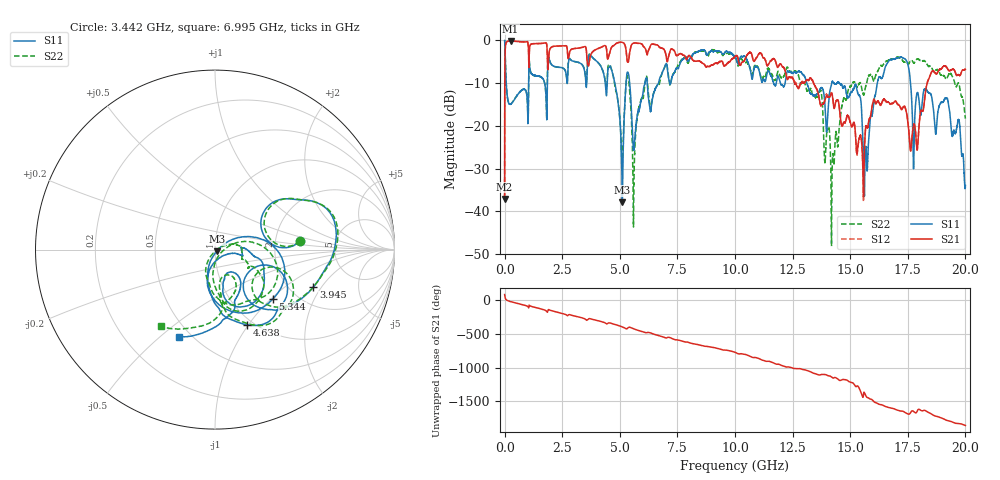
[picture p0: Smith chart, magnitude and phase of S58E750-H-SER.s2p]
!{S58E750}
!Johanson Technology Inc.
!www.johansontechnology.com
!Test Board Conditions:
!Substrate Type  RO4350B
!Substrate Thickness  60 mil
!Substrate Dk  3.66
!TL Type: GCPW
!TL Trace Width  115 mil
!TL Gap  52 mil
!Electrode orientation  Horizontal
!DUT TOPOLOGY	SERIES
!Mounting Pad LxW  55x428 mil
! Created Wed Apr 14 12:01:42 2021
# mhz S ma R 50
! 2 Port Network Data from SP1.SP block
! freq  magS11  angS11  magS21  angS21  magS12  angS12  magS22  angS22
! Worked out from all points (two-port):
!   20001 points, 300 kHz to 20 GHz, reference 50 ohm
!   highest |S21| = -0.15 dB at 256.3 MHz (marker M1); lowest = -37.2 dB at 300 kHz (marker M2)
!   |S21| within 3 dB of the highest: 21.1 MHz to 1.042 GHz (1.021 GHz wide, 192 % of centre); 1.925 GHz to 2.731 GHz (805.9 MHz wide, 34.6 % of centre)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
!   lowest |S11| = -37.9 dB at 5.11 GHz (marker M3), VSWR 1.03, Z = 51 - j0.854 ohm
!   |S11| at or under -10 dB: 13.12 GHz to 14.2 GHz (1.082 GHz wide, 7.92 % of centre); 14.54 GHz to 16.18 GHz (1.641 GHz wide, 10.7 % of centre); 17.62 GHz to end of sweep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
!   |S22| runs from -48.2 to 0.0 dB; largest |S21 - S12| = 0.016
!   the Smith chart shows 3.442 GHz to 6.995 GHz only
!   S11 on the Smith chart (normalised r, x): 3.442 GHz: 2.75, +0.35; 3.945 GHz: 2.64, -1.69; 4.638 GHz: 0.93, -0.99; 5.344 GHz: 1.54, -1.03; 6.995 GHz: 0.43, -0.58
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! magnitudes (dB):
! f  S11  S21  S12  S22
! 300 kHz  0.0  -37.2  -37.1  -0.1
! 104.3 MHz  -12.5  -0.3  -0.3  -12.5
! 256.3 MHz  -15.0  -0.1  -0.2  -14.9
! 3.334 GHz  -5.5  -1.7  -1.7  -5.5
! 3.442 GHz  -6.5  -1.5  -1.5  -6.4
! 3.945 GHz  -4.6  -2.2  -2.2  -4.6
! 4.638 GHz  -6.8  -1.7  -1.7  -6.8
! 5.11 GHz  -37.9  -0.5  -0.5  -28.8
! 5.344 GHz  -7.5  -5.1  -5.1  -8.9
! 5.617 GHz  -25.3  -0.6  -0.6  -31.9
! 6.107 GHz  -9.6  -1.9  -1.9  -9.6
! 6.667 GHz  -10.2  -1.2  -1.2  -10.4
! 6.995 GHz  -5.6  -3.2  -3.2  -5.6
! 10 GHz  -3.8  -3.8  -3.8  -3.8
! 13.33 GHz  -12.5  -9.1  -9.3  -12.1
! 14.23 GHz  -9.5  -13.2  -13.1  -27.2
! 15.31 GHz  -12.0  -25.9  -26.4  -10.9
! 15.68 GHz  -24.9  -20.3  -20.4  -10.7
! 16.67 GHz  -4.9  -14.5  -14.7  -4.6
! 17.9 GHz  -12.4  -25.5  -25.5  -4.4
! 19.18 GHz  -13.6  -6.3  -6.3  -9.0
! 20 GHz  -34.0  -6.8  -6.7  -18.3
